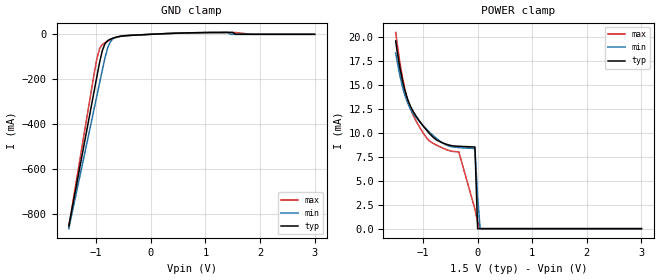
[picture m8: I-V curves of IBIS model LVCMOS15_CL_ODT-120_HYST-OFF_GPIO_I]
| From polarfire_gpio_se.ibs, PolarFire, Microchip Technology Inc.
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|   Model LVCMOS15_CL_ODT-120_HYST-OFF_GPIO_I
[Model]   LVCMOS15_CL_ODT-120_HYST-OFF_GPIO_I
Model_type   Input
Vinl =   0.525
Vinh =   0.975
|   typ   min   max
C_comp_pullup   2.605e-12   2.605e-12   2.76e-12
C_comp_pulldown  2.605e-12   2.605e-12   2.76e-12
[Temperature Range]  25C   100C   -40C
[Voltage Range]  1.5   1.425   1.575
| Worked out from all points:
|   GND clamp passes 1 mA (typ) near -0.08 V on its own axis
|   POWER clamp passes 1 mA (typ) near -0.01 V on its own axis
[GND Clamp]
| Voltage   I(typ)   I(min)   I(max)
-1.5V     -852.5mA   -863.7mA   -854.8mA
-984.4mV  -185.7mA   -271mA     -105.6mA
-935.2mV  -123.6mA   -214.5mA   -62.78mA
-885.9mV  -71.93mA   -158.1mA   -45.72mA
-836.7mV  -41.29mA   -103.4mA   -37.18mA
-787.5mV  -28.06mA   -59.45mA   -30.09mA
-738.3mV  -21.49mA   -32.42mA   -23.67mA
-689.1mV  -16.88mA   -19.73mA   -18.12mA
-541.4mV  -8.34mA    -8.6mA     -7.922mA
1.078V    8.054mA    7.928mA    7.536mA
1.453V    8.469mA    0A         7.897mA
3V        0A         0A         0A
[POWER Clamp]
| Voltage   I(typ)   I(min)   I(max)
-1.5V     19.54mA    18.27mA    20.43mA
-1.378V   15.46mA    14.81mA    15.8mA
-1.28V    13.45mA    13.06mA    13.32mA
-1.181V   12.21mA    12mA       11.82mA
-1.034V   10.97mA    10.94mA    10.29mA
-885.9mV  9.934mA    10.07mA    9.158mA
-738.3mV  9.186mA    9.325mA    8.659mA
-344.5mV  8.573mA    8.438mA    7.999mA
-49.22mV  8.503mA    8.34mA     2.028mA
0V        0A         3.333mA    697.2uA
46.88mV   0A         0A         0A
3V        0A         0A         0A
